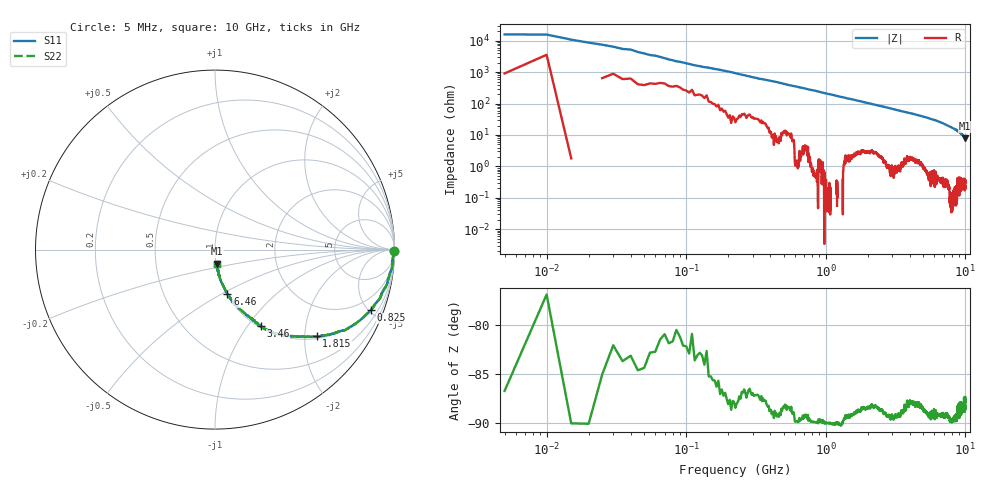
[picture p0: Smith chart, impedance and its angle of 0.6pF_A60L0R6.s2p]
! Amotech Co.,Ltd.
! http://www.amotech.co.kr/
! Part Number: A60L0R6
! These Parameters are Measured in Series Mode Connection
! Operation Temp=25[degC], DC Bias Voltage=0[V]
! Freq. Start=5[MHz] Stop=10[GHz], 2000[Steps]
! Date: Monday, July 14, 2020, 09:26:03
# GHZ S RI R 50.000000
!Freq.(Hz) S11(Real) S11(Imag) S21(Real) S21(Imag) S12(Real) S12(Imag) S22(Real) S22(Imag)
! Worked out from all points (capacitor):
!   2000 points, 5 MHz to 10 GHz, reference 50 ohm
!   read as one part in series: C = 846 fF near 55 MHz
!   lowest |Z| = 7.92 ohm at 9.99 GHz (marker M1)
!   S11 on the Smith chart (normalised r, x): 5 MHz: open; 825 MHz: 1.01, -5.15; 1.815 GHz: 1.06, -2.29; 3.46 GHz: 1.02, -1.16; 6.46 GHz: 1.01, -0.53; 10 GHz: 1.00, -0.16
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0.005  0.9996 -0.00638  0.00041 0.00638  0.00041 0.00638  0.9996 -0.00638
0.03  0.9976 -0.0154  0.0024 0.0154  0.0024 0.0154  0.9976 -0.0154
0.07  0.993 -0.0354  0.00697 0.0354  0.00697 0.0354  0.993 -0.0354
0.1  0.9902 -0.0513  0.0098 0.0513  0.0098 0.0513  0.9902 -0.0513
0.145  0.9889 -0.0712  0.0111 0.0712  0.0111 0.0712  0.9889 -0.0712
0.225  0.9854 -0.107  0.0146 0.107  0.0146 0.107  0.9854 -0.107
0.33  0.9676 -0.1542  0.0324 0.1542  0.0324 0.1542  0.9676 -0.1542
0.5  0.9413 -0.2203  0.0587 0.2203  0.0587 0.2203  0.9413 -0.2203
0.825  0.8681 -0.3371  0.1319 0.3371  0.1319 0.3371  0.8681 -0.3371
1.235  0.7399 -0.438  0.2601 0.438  0.2601 0.438  0.7399 -0.438
1.675  0.6046 -0.4787  0.3954 0.4787  0.3954 0.4787  0.6046 -0.4787
1.815  0.5658 -0.4829  0.4342 0.4829  0.4342 0.4829  0.5658 -0.4829
2.515  0.4015 -0.4779  0.5985 0.4779  0.5985 0.4779  0.4015 -0.4779
3.34  0.2667 -0.4343  0.7333 0.4343  0.7333 0.4343  0.2667 -0.4343
3.46  0.2548 -0.4263  0.7452 0.4263  0.7452 0.4263  0.2548 -0.4263
5.005  0.1336 -0.3283  0.8664 0.3283  0.8664 0.3283  0.1336 -0.3283
6.46  0.0695 -0.2464  0.9305 0.2464  0.9305 0.2464  0.0695 -0.2464
6.67  0.062 -0.235  0.938 0.235  0.938 0.235  0.062 -0.235
8.335  0.0245 -0.1524  0.9755 0.1524  0.9755 0.1524  0.0245 -0.1524
9.24  0.0154 -0.1137  0.9846 0.1137  0.9846 0.1137  0.0154 -0.1137
9.99  0.00855 -0.0783  0.9914 0.0783  0.9914 0.0783  0.00855 -0.0783
10  0.00861 -0.0787  0.9914 0.0787  0.9914 0.0787  0.00861 -0.0787
